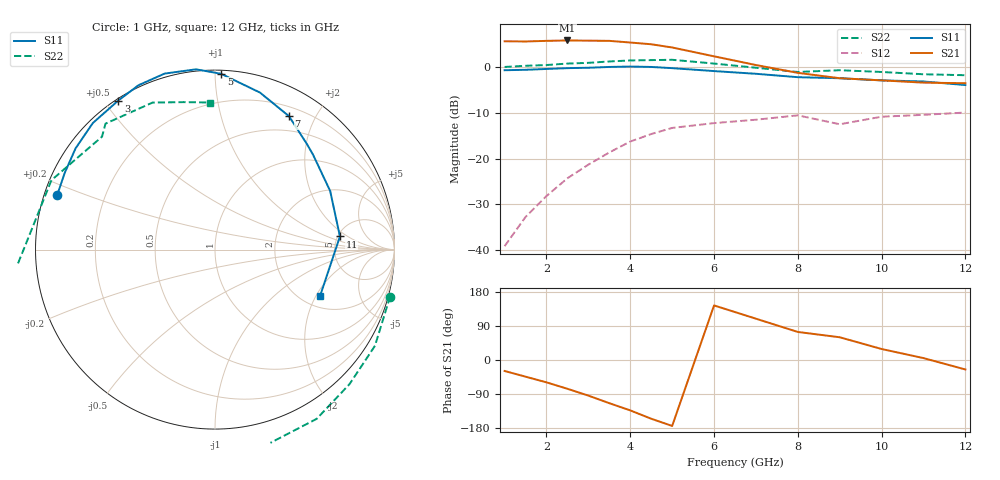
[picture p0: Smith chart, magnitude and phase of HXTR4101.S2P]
! HXTR-4101 Common Base
! Vce=15V  Ic=30mA
# ghz s ma r 50
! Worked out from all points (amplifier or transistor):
!   16 points, 1 GHz to 12 GHz, reference 50 ohm
!   highest |S21| = 5.9 dB at 2.5 GHz (marker M1)
!   |S21| within 3 dB of that: start of sweep to 5.753 GHz
!   unconditionally stable (mu >= 1): 11.82 GHz to end of sweep
!   at 2 GHz: K = -0.83, MSG = 17.0 dB, |S12| = -28.2 dB
!   at 5 GHz: K = -0.42, MSG = 8.8 dB, |S12| = -13.3 dB
!   at 12 GHz: K = 1.02, MAG = 2.4 dB, |S12| = -9.9 dB
!   S11 on the Smith chart (normalised r, x): 1 GHz: 0.04, +0.17; 3 GHz: 0.01, +0.54; 5 GHz: 0.02, +1.04; 7 GHz: 0.31, +1.66; 11 GHz: 5.22, +1.50; 12 GHz: 2.46, -2.17
1  0.93 161.0  1.93 -29.0  0.011 127.0  1.01 -15.0
1.5  0.94 153.0  1.92 -44.0  0.023 126.0  1.04 -31.0
2  0.96 144.0  1.95 -59.0  0.039 120.0  1.06 -45.0
2.5  0.98 134.0  1.97 -76.0  0.061 113.0  1.1 -59.0
3  0.99 123.0  1.96 -94.0  0.086 105.0  1.12 -74.0
3.5  1.01 115.0  1.95 -114.0  0.117 93.0  1.16 -91.0
4  1.02 106.0  1.87 -133.0  0.154 84.0  1.19 -108.0
4.5  1.01 96.0  1.79 -155.0  0.186 70.0  1.2 -127.0
5  0.98 88.0  1.65 -174.0  0.217 58.0  1.21 -143.0
6  0.91 74.0  1.32 144.0  0.245 35.0  1.1 -176.0
7  0.85 61.0  1.06 109.0  0.267 17.0  0.99 157.0
8  0.78 49.0  0.87 74.0  0.298 1.0  0.89 135.0
9  0.76 44.0  0.76 60.0  0.238 -10.0  0.93 131.0
10  0.72 27.0  0.72 29.0  0.288 -24.0  0.89 113.0
11  0.7 6.0  0.68 5.0  0.302 -38.0  0.84 102.0
12  0.64 -24.0  0.67 -25.0  0.32 -58.0  0.82 92.0
